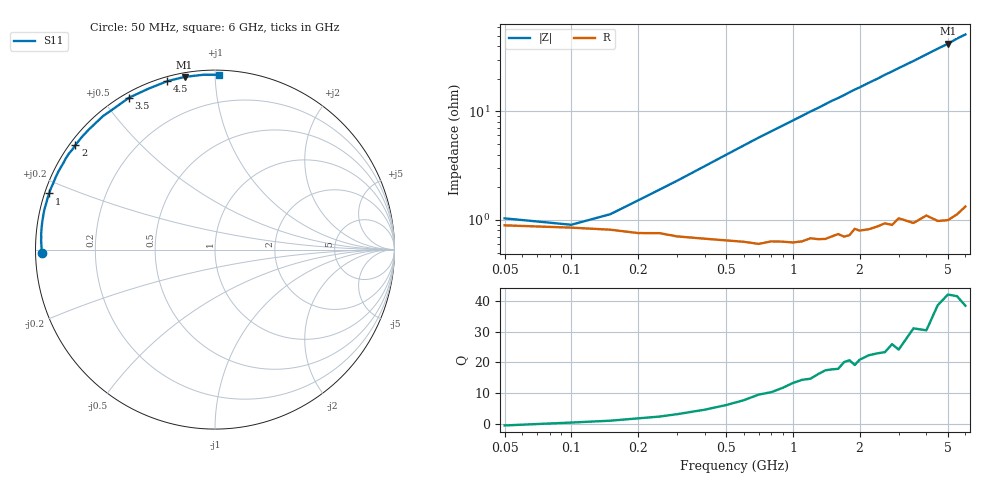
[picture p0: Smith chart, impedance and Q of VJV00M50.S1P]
! Infineon Technologies  Discrete & RF Semiconductors
! BB 914
! Si Tuning Diode in SOT23
! VR =
! S-Parameters:  July  1999
# GHz  S  MA  R  50
!  f  S11
! GHz  MAG  ANG
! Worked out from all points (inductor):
!   34 points, 50 MHz to 6 GHz, reference 50 ohm
!   read as one part to ground: L = 1.22 nH near 300 MHz
!   highest Q = 41.6 at 5 GHz (marker M1), where L = 1.34 nH
!   S11 on the Smith chart (normalised r, x): 50 MHz: 0.02, -0.01; 1 GHz: 0.01, +0.16; 2 GHz: 0.02, +0.33; 3.5 GHz: 0.02, +0.58; 4.5 GHz: 0.02, +0.76; 6 GHz: 0.03, +1.02
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0.05  0.965 -178.8
0.1  0.9666 179.3
0.2  0.9702 177.0
0.3  0.9722 175.0
0.5  0.9746 171.0
0.7  0.9766 167.0
0.8  0.9754 165.1
1  0.9762 161.3
1.2  0.9743 157.5
1.3  0.9749 155.7
1.4  0.975 153.8
1.5  0.9738 151.9
1.6  0.9727 150.3
1.7  0.9743 148.5
1.8  0.9738 146.6
1.9  0.9704 144.8
2  0.9717 143.2
2.2  0.9715 139.7
2.4  0.9705 136.5
2.6  0.9692 133.0
2.8  0.9709 130.0
3  0.9674 126.8
3.5  0.9724 119.5
4  0.9701 112.4
4.5  0.9754 105.8
5  0.9769 100.0
5.5  0.9763 93.7
6  0.9744 88.7
